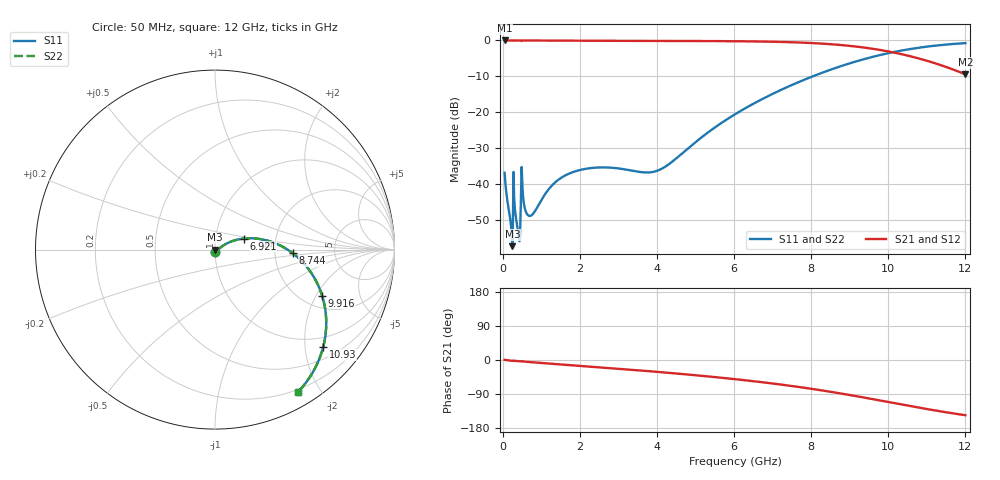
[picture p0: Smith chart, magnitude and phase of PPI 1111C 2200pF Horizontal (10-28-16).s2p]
# MHz S MA R 50
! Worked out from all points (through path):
!   1601 points, 50 MHz to 12 GHz, reference 50 ohm
!   highest |S21| = 0.00 dB at 57.47 MHz (marker M1); lowest = -9.4 dB at 12 GHz (marker M2)
!   group delay of S21, straight-line fit = 33.3 ps
!   lowest |S11| = -57.4 dB at 251.7 MHz (marker M3), VSWR 1.00, Z = 50.1 - j0.0565 ohm
!   |S11| at or under -10 dB: start of sweep to 8.043 GHz
!   |S22| runs from -57.4 to -0.7 dB; largest |S21 - S12| = 0
!   S11 on the Smith chart (normalised r, x): 50 MHz: 1.00, -0.03; 6.921 GHz: 1.37, +0.17; 8.744 GHz: 2.52, -0.12; 9.916 GHz: 2.53, -2.24; 10.93 GHz: 0.76, -2.40; 12 GHz: 0.17, -1.73
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50  0.01435 -88.1  0.9995 0.4  0.9995 0.4  0.01435 -88.1
57.46875  0.01248 -88.0  0.9995 0.3  0.9995 0.3  0.01248 -88.0
199.375  0.003118 -78.6  0.9993 -1.4  0.9993 -1.4  0.003118 -78.6
251.6562  0.001356 -24.6  0.9987 -2.0  0.9987 -2.0  0.001356 -24.6
326.3438  0.003964 -78.4  0.999 -2.4  0.999 -2.4  0.003964 -78.4
371.1562  0.002714 -71.4  0.999 -2.8  0.999 -2.8  0.002714 -71.4
401.0312  0.002105 -60.9  0.9989 -3.1  0.9989 -3.1  0.002105 -60.9
498.125  0.01484 -49.5  0.9896 -3.4  0.9896 -3.4  0.01484 -49.5
528  0.006794 -75.1  0.9978 -3.8  0.9978 -3.8  0.006794 -75.1
610.1562  0.003993 -68.4  0.9982 -4.7  0.9982 -4.7  0.003993 -68.4
729.6562  0.00361 -51.3  0.9974 -5.7  0.9974 -5.7  0.00361 -51.3
1357.031  0.01046 -38.4  0.9907 -10.5  0.9907 -10.5  0.01046 -38.4
2044.156  0.01582 -56.0  0.9878 -15.6  0.9878 -15.6  0.01582 -56.0
4038.312  0.01548 -15.4  0.9849 -31.5  0.9849 -31.5  0.01548 -15.4
6025  0.09346 27.0  0.9753 -50.6  0.9753 -50.6  0.09346 27.0
6921.25  0.1714 21.0  0.9611 -61.0  0.9611 -61.0  0.1714 21.0
8019.156  0.3126 8.2  0.9196 -76.2  0.9196 -76.2  0.3126 8.2
8743.625  0.4331 -2.6  0.8662 -87.9  0.8662 -87.9  0.4331 -2.6
9916.219  0.6493 -23.2  0.7166 -109.3  0.7166 -109.3  0.6493 -23.2
10013.31  0.6666 -25.0  0.7008 -111.1  0.7008 -111.1  0.6666 -25.0
10931.97  0.8106 -41.9  0.5343 -128.2  0.5343 -128.2  0.8106 -41.9
12000  0.9179 -59.7  0.3371 -145.7  0.3371 -145.7  0.9179 -59.7
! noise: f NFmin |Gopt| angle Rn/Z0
50  0.0004112  0.878  0.4054  0.0007287
1372  0.01095  0.8755  10.9  0.01881
2701  0.0179  0.8551  21.26  0.02549
4031  0.02303  0.8396  31.24  0.02822
5360  0.02857  0.8367  40.72  0.03254
6682  0.03517  0.8436  49.54  0.03941
8012  0.04387  0.8584  57.79  0.05088
9341  0.05633  0.8792  65.41  0.07157
1.067e+04  0.07641  0.9047  72.46  0.1146
1.2e+04  0.1151  0.9335  78.99  0.2296
